[IBIS Ver]   4.2
[File Name]  stm32f2_lqfp176.ibs
[File Rev]   1.0
[Date]   31-Aug-2011
[Source]   STMicroelectronics NV
[Notes]   The I/O models have been made by simulation and qualified
   with recomandation of QualityIBIS flow.
   Some Models, library and pin names may be modified.
   Details of modified names can be found below.
ORIGINAL NAME   ::  MODIFIED NAME   :: COMMENTS(if any)
IO8USB_LSFS_OTG_FT  ::  IO8USB_LSFS_OTG_FT_USB   :: Model in USB mode.
IO8USB_LSFS_OTG_FT  ::  IO8USB_LSFS_OTG_FT_NON_USB_DNV33  :: Model in other than USB mode & pad pin = DNV33
IO8USB_LSFS_OTG_FT  ::  IO8USB_LSFS_OTG_FT_NON_USB_DPV33  :: Model in other than USB mode & pad pin = DPV33
[Disclaimer] These IBIS models are the proprietary information of
   STMicroelectronics and are disclosed to users solely for
   modeling and simulation purposes. No further license is
   implied. All warranties express, implied, or statutory,
   including any implied warranty of fitness for a particular
   purpose or implied warranty against infringement, are
   hereby disclaimed. STMicroelectronics reserves the right
   to change the IBIS models at any time and without notice.
[Copyright]  (c) STMicroelectronics
   All rights reserved. Reproduction in whole or part is prohibited
   without the written consent of the copyright holder.
[Component]  STM32F2_LQFP176
[Manufacturer] STMicroelectronics NV
[Package]
| variable   typ   min   max
R_pkg   0.000mOhm   0.000mOhm   0.000mOhm
L_pkg   0.000nH   0.000nH   0.000nH
C_pkg   0.000pF   0.000pF   0.000pF
[Pin]   signal_name   model_name
1 PE2 IO8PROG2M25M50M100M_ARSUDQ_FT
2 PE3 IO8PROG2M25M50M100M_ARSUDQ_FT
3 PE4 IO8PROG2M25M50M100M_ARSUDQ_FT
4 PE5 IO8PROG2M25M50M100M_ARSUDQ_FT
5 PE6 IO8PROG2M25M50M100M_ARSUDQ_FT
|6 VBAT VDD33IOSWCO_MOSSWI_FT
7 PI8 IO8PROG2M25M50M100M_ARSUDQ_FT_V33
8 PC13 IO8PROG2M25M50M100M_ARWSUDQ_FT_V33
9 PC14 IO8PROG2M25M50M100M_ARWSUDQ_FT
10 PC15 IO8PROG2M25M50M100M_ARSUDQ_FT
11 PI9  IO8PROG2M25M50M100M_ARSUDQ_FT
12 PI10 IO8PROG2M25M50M100M_ARSUDQ_FT
13 PI11 IO8PROG2M25M50M100M_ARSUDQ_FT
|14 VSS_13 VSSIOCO
|15 VDD_13 VDD33IOCO
16 PF0 IO8PROG2M25M50M100M_ARSUDQ_FT
17 PF1 IO8PROG2M25M50M100M_ARSUDQ_FT
18 PF2 IO8PROG2M25M50M100M_ARSUDQ_FT
19 PF3 IO8PROG2M25M50M100M_ARSUDQ_FT
20 PF4 IO8PROG2M25M50M100M_ARSUDQ_FT
21 PF5 IO8PROG2M25M50M100M_ARSUDQ_FT
|22 VSS_5 VSSIOCO
|23 VDD_5 VDD33IOCO
24 PF6 IO8PROG2M25M50M100M_ARSUDQ_FT
25 PF7 IO8PROG2M25M50M100M_ARSUDQ_FT
26 PF8 IO8PROG2M25M50M100M_ARSUDQ_FT
27 PF9  IO8PROG2M25M50M100M_AR3WSUDQ_FT
28 PF10 IO8PROG2M25M50M100M_ARSUDQ_FT
29 PH0 IO8PROG2M25M50M100M_ARSUDQ_FT
30 PH1 IO8PROG2M25M50M100M_ARSUDQ_FT
|31 NRST RESET
32 PC0 IO8PROG2M25M50M100M_AR3WSUDQ_FT
33 PC1 IO8PROG2M25M50M100M_AR3WSUDQ_FT
34 PC2 IO8PROG2M25M50M100M_AR3WSUDQ_FT
35 PC3 IO8PROG2M25M50M100M_AR3WSUDQ_FT
|36 VDD_12 VDD33IOCO_VSSIOCO_MOSSWI_FT
|37 VSSA VSSCO
|38 VREF+ VDD33CO
|39 VDDA VDD33CO
40 PA0 IO8PROG2M25M50M100M_AR3WSUDQ_FT_V33
41 PA1 IO8PROG2M25M50M100M_AR3WSUDQ_FT
42 PA2 IO8PROG2M25M50M100M_AR3WSUDQ_FT
43 PH2 IO8PROG2M25M50M100M_AR3WSUDQ_FT
44 PH3 IO8PROG2M25M50M100M_AR3WSUDQ_FT
45 PH4 IO8PROG2M25M50M100M_AR3WSUDQ_FT
46 PH5 IO8PROG2M25M50M100M_AR3WSUDQ_FT
47 PA3 IO8PROG2M25M50M100M_AR3WSUDQ_FT
|48 VSS_4 VSSIOCO
|49 VDD_4 VDD33IOCO
50 PA4 IO8PROG2M25M50M100M_AR3WSUDQ_FT
51 PA5 IO8PROG2M25M50M100M_AR3WSUDQ_FT
52 PA6 IO8PROG2M25M50M100M_AR3WSUDQ_FT
53 PA7 IO8PROG2M25M50M100M_AR3WSUDQ_FT
54 PC4 IO8PROG2M25M50M100M_AR3WSUDQ_FT
55 PC5 IO8PROG2M25M50M100M_AR3WSUDQ_FT
56 PB0 IO8PROG2M25M50M100M_AR3WSUDQ_FT
57 PB1 IO8PROG2M25M50M100M_AR3WSUDQ_FT
58 PB2 IO8PROG2M25M50M100M_AR3WSUDQ_FT
59 PF11 IO8PROG2M25M50M100M_ARSUDQ_FT
60 PF12 IO8PROG2M25M50M100M_ARSUDQ_FT
|61 VSS_6 VSSIOCO
|62 VDD_6 VDD33IOCO
63 PF13 IO8PROG2M25M50M100M_ARSUDQ_FT
64 PF14 IO8PROG2M25M50M100M_ARSUDQ_FT
65 PF15 IO8PROG2M25M50M100M_ARSUDQ_FT
66 PG0 IO8PROG2M25M50M100M_ARSUDQ_FT
67 PG1 IO8PROG2M25M50M100M_ARSUDQ_FT
68 PE7 IO8PROG2M25M50M100M_ARSUDQ_FT
69 PE8 IO8PROG2M25M50M100M_ARSUDQ_FT
70 PE9 IO8PROG2M25M50M100M_ARSUDQ_FT
|71 VSS_7 VSSIOCO
|72 VDD_7 VDD33IOCO
73 PE10 IO8PROG2M25M50M100M_ARSUDQ_FT
74 PE11 IO8PROG2M25M50M100M_ARSUDQ_FT
75 PE12 IO8PROG2M25M50M100M_ARSUDQ_FT
76 PE13 IO8PROG2M25M50M100M_ARSUDQ_FT
77 PE14 IO8PROG2M25M50M100M_ARSUDQ_FT
78 PE15 IO8PROG2M25M50M100M_ARSUDQ_FT
79 PB10 IO8PROG2M25M50M100M_ARSUDQ_I2CIN_FT
80 PB11 IO8PROG2M25M50M100M_ARSUDQ_I2CIN_FT
|81 VCAP_1
|82 VDD_1 VDD33IOCO
83 PH6 IO8PROG2M25M50M100M_ARSUDQ_FT
84 PH7 IO8PROG2M25M50M100M_ARSUDQ_FT
85 PH8 IO8PROG2M25M50M100M_ARSUDQ_FT
86 PH9 IO8PROG2M25M50M100M_ARSUDQ_FT
87 PH10 IO8PROG2M25M50M100M_ARSUDQ_FT
88 PH11 IO8PROG2M25M50M100M_ARSUDQ_FT
89 PH12 IO8PROG2M25M50M100M_ARSUDQ_FT
|90 VSS_14 VSSIOCO
|91 VDD_14 VDD33IOCO
92 PB12 IO8USB_ID_OTG_FT
93 PB13 IO8USB_VBUS_OTG_FT
94 PB14 IO8USB_LSFS_OTG_FT_USB
|94 PB14 IO8USB_LSFS_OTG_FT_NON_USB_DNV33
95 PB15 IO8USB_LSFS_OTG_FT_USB
|95 PB15 IO8USB_LSFS_OTG_FT_NON_USB_DPV3394
96 PD8 IO8PROG2M25M50M100M_ARSUDQ_FT
97 PD9 IO8PROG2M25M50M100M_ARSUDQ_FT
98 PD10 IO8PROG2M25M50M100M_ARSUDQ_FT
99 PD11 IO8PROG2M25M50M100M_ARSUDQ_FT
100 PD12 IO8PROG2M25M50M100M_ARSUDQ_FT
101 PD13 IO8PROG2M25M50M100M_ARSUDQ_FT
|102 VSS_8 VSSIOCO
|103 VDD_8 VDD33IOCO
104 PD14 IO8PROG2M25M50M100M_ARSUDQ_FT
105 PD15 IO8PROG2M25M50M100M_ARSUDQ_FT
106 PG2 IO8PROG2M25M50M100M_ARSUDQ_FT
107 PG3 IO8PROG2M25M50M100M_ARSUDQ_FT
108 PG4 IO8PROG2M25M50M100M_ARSUDQ_FT
109 PG5 IO8PROG2M25M50M100M_ARSUDQ_FT
110 PG6 IO8PROG2M25M50M100M_ARSUDQ_FT
111 PG7 IO8PROG2M25M50M100M_ARSUDQ_FT
112 PG8 IO8PROG2M25M50M100M_ARSUDQ_FT
|113 VSS_9 VSSIOCO
|114 VDD_9 VDD33IOCO
115 PC6 IO8PROG2M25M50M100M_ARSUDQ_FT
116 PC7 IO8PROG2M25M50M100M_ARSUDQ_FT
117 PC8 IO8PROG2M25M50M100M_ARSUDQ_FT
118 PC9 IO8PROG2M25M50M100M_ARSUDQ_I2CIN_FT
119 PA8 IO8PROG2M25M50M100M_ARSUDQ_I2CIN_FT
120 PA9 IO8USB_VBUS_OTG_FT
121 PA10 IO8USB_ID_OTG_FT
|122 PA11 IO8USB_LSFS_OTG_FT_USB
122 PA11 IO8USB_LSFS_OTG_FT_NON_USB_DNV33
|123 PA12 IO8USB_LSFS_OTG_FT_USB
123 PA12 IO8USB_LSFS_OTG_FT_NON_USB_DPV33
124 PA13 IO8PROG2M25M50M100M_ARSUDQ_FT
|125 VCAP_2
|126 VSS_2 VSSIOCO
|127 VDD_2 VDD33IOCO
128 PH13 IO8PROG2M25M50M100M_ARSUDQ_FT
129 PH14 IO8PROG2M25M50M100M_ARSUDQ_FT
130 PH15 IO8PROG2M25M50M100M_ARSUDQ_FT
131 PI0 IO8PROG2M25M50M100M_ARSUDQ_FT
132 PI1 IO8PROG2M25M50M100M_ARSUDQ_FT
133 PI2 IO8PROG2M25M50M100M_ARSUDQ_FT
134 PI3 IO8PROG2M25M50M100M_ARSUDQ_FT
|135 VSS_15 VSSIOCO
|136 VDD_15 VDD33IOCO
137 PA14 IO8PROG2M25M50M100M_ARSUDQ_FT
138 PA15 IO8PROG2M25M50M100M_AR3WSUDQ_FT
139 PC10 IO8PROG2M25M50M100M_ARSUDQ_FT
140 PC11 IO8PROG2M25M50M100M_ARSUDQ_FT
141 PC12 IO8PROG2M25M50M100M_ARSUDQ_FT
142 PD0 IO8PROG2M25M50M100M_ARSUDQ_FT
143 PD1 IO8PROG2M25M50M100M_ARSUDQ_FT
144 PD2 IO8PROG2M25M50M100M_ARSUDQ_FT
145 PD3 IO8PROG2M25M50M100M_ARSUDQ_FT
146 PD4 IO8PROG2M25M50M100M_ARSUDQ_FT
147 PD5 IO8PROG2M25M50M100M_ARSUDQ_FT
|148 VSS_10 VSSIOCO
|149 VDD_10 VDD33IOCO
150 PD6 IO8PROG2M25M50M100M_ARSUDQ_FT
151 PD7 IO8PROG2M25M50M100M_ARSUDQ_FT
152 PG9 IO8PROG2M25M50M100M_ARSUDQ_FT
153 PG10 IO8PROG2M25M50M100M_ARSUDQ_FT
154 PG11 IO8PROG2M25M50M100M_ARSUDQ_FT
155 PG12 IO8PROG2M25M50M100M_ARSUDQ_FT
156 PG13 IO8PROG2M25M50M100M_ARSUDQ_FT
157 PG14 IO8PROG2M25M50M100M_ARSUDQ_FT
|158 VSS_11 VSSIOCO
|159 VDD_11 VDD33IOCO
160 PG15 IO8PROG2M25M50M100M_ARSUDQ_FT
161 PB3 IO8PROG2M25M50M100M_ARSUDQ_FT
162 PB4 IO8PROG2M25M50M100M_ARSUDQ_FT
163 PB5 IO8PROG2M25M50M100M_AR3WSUDQ_FT
164 PB6 IO8PROG2M25M50M100M_ARSUDQ_I2CIN_FT
165 PB7 IO8PROG2M25M50M100M_ARSUDQ_I2CIN_FT
166 BOOT0 VPP_TEST_HV
167 PB8 IO8PROG2M25M50M100M_ARSUDQ_I2CIN_FT
168 PB9 IO8PROG2M25M50M100M_ARSUDQ_I2CIN_FT
169 PE0 IO8PROG2M25M50M100M_ARSUDQ_FT
170 PE1 IO8PROG2M25M50M100M_ARSUDQ_FT
|171 VSS VSSIOCO
|172 VDD_3 VDD33IOCO
173 PI4 IO8PROG2M25M50M100M_ARSUDQ_FT
174 PI5 IO8PROG2M25M50M100M_ARSUDQ_FT
175 PI6 IO8PROG2M25M50M100M_ARSUDQ_FT
176 PI7 IO8PROG2M25M50M100M_ARSUDQ_FT
[Diff Pin]  inv_pin   vdiff tdelay_typ tdelay_min tdelay_max
94 95 200mV 0  0 0
122 123 200mV 0  0 0
[Model Selector] IO8PROG2M25M50M100M_ARSUDQ_FT_V33
IO8PROG2M25M50M100M_ARSUDQ_DRV_V33_00   DRIVER MODEL  : SPEEDAV33=0 SPEEDBV33=0
IO8PROG2M25M50M100M_ARSUDQ_DRV_V33_01   DRIVER MODEL  : SPEEDAV33=0 SPEEDBV33=1
IO8PROG2M25M50M100M_ARSUDQ_DRV_V33_10   DRIVER MODEL  : SPEEDAV33=1 SPEEDBV33=0
IO8PROG2M25M50M100M_ARSUDQ_DRV_V33_11   DRIVER MODEL  : SPEEDAV33=1 SPEEDBV33=1
IO8PROG2M25M50M100M_ARSUDQ_RCV_V33_0   CMOS RECIEVER : ENHYSV33=0  OUTPUT=ZIV33
IO8PROG2M25M50M100M_ARSUDQ_RCV_V33_0_T   TTL  RECIEVER : ENHYSV33=0  OUTPUT=ZIV33
IO8PROG2M25M50M100M_ARSUDQ_RCV_V33_1   CMOS RECIEVER : ENHYSV33=1  OUTPUT=ZIV33
IO8PROG2M25M50M100M_ARSUDQ_RCV_V33_1_T   TTL  RECIEVER : ENHYSV33=1  OUTPUT=ZIV33
[Model Selector] IO8PROG2M25M50M100M_AR3WSUDQ_FT_V33
IO8PROG2M25M50M100M_AR3WSUDQ_DRV_V33_00   DRIVER MODEL  : SPEEDAV33=0 SPEEDBV33=0
IO8PROG2M25M50M100M_AR3WSUDQ_DRV_V33_01   DRIVER MODEL  : SPEEDAV33=0 SPEEDBV33=1
IO8PROG2M25M50M100M_AR3WSUDQ_DRV_V33_10   DRIVER MODEL  : SPEEDAV33=1 SPEEDBV33=0
IO8PROG2M25M50M100M_AR3WSUDQ_DRV_V33_11   DRIVER MODEL  : SPEEDAV33=1 SPEEDBV33=1
IO8PROG2M25M50M100M_AR3WSUDQ_RCV_V33_0   CMOS RECIEVER : ENHYSV33=0  OUTPUT=ZIV33
IO8PROG2M25M50M100M_AR3WSUDQ_RCV_V33_0_T  TTL  RECIEVER : ENHYSV33=0  OUTPUT=ZIV33
IO8PROG2M25M50M100M_AR3WSUDQ_RCV_V33_1   CMOS RECIEVER : ENHYSV33=1  OUTPUT=ZIV33
IO8PROG2M25M50M100M_AR3WSUDQ_RCV_V33_1_T  TTL  RECIEVER : ENHYSV33=1  OUTPUT=ZIV33
[Model Selector] IO8PROG2M25M50M100M_AR3WSUDQ_FT
IO8PROG2M25M50M100M_AR3WSUDQ_FT_DRV_00   DRIVER MODEL  : SPEEDAV12=0 SPEEDBV12=0
IO8PROG2M25M50M100M_AR3WSUDQ_FT_DRV_01   DRIVER MODEL  : SPEEDAV12=0 SPEEDBV12=1
IO8PROG2M25M50M100M_AR3WSUDQ_FT_DRV_10   DRIVER MODEL  : SPEEDAV12=1 SPEEDBV12=0
IO8PROG2M25M50M100M_AR3WSUDQ_FT_DRV_11   DRIVER MODEL  : SPEEDAV12=1 SPEEDBV12=1
IO8PROG2M25M50M100M_AR3WSUDQ_FT_RCV_00   CMOS RECIEVER : ENHYSV12=0  OUTPUT=ZIV12
IO8PROG2M25M50M100M_AR3WSUDQ_FT_RCV_00_T  TTL  RECIEVER : ENHYSV12=0  OUTPUT=ZIV12
IO8PROG2M25M50M100M_AR3WSUDQ_FT_RCV_01   CMOS RECIEVER : ENHYSV12=0  OUTPUT=ZIV33
IO8PROG2M25M50M100M_AR3WSUDQ_FT_RCV_01_T  TTL  RECIEVER : ENHYSV12=0  OUTPUT=ZIV33
IO8PROG2M25M50M100M_AR3WSUDQ_FT_RCV_10   CMOS RECIEVER : ENHYSV12=1  OUTPUT=ZIV12
IO8PROG2M25M50M100M_AR3WSUDQ_FT_RCV_10_T  TTL  RECIEVER : ENHYSV12=1  OUTPUT=ZIV12
IO8PROG2M25M50M100M_AR3WSUDQ_FT_RCV_11   CMOS RECIEVER : ENHYSV12=1  OUTPUT=ZIV33
IO8PROG2M25M50M100M_AR3WSUDQ_FT_RCV_11_T  TTL  RECIEVER : ENHYSV12=1  OUTPUT=ZIV33
[Model Selector] IO8PROG2M25M50M100M_ARSUDQ_FT
IO8PROG2M25M50M100M_ARSUDQ_FT_DRV_00   DRIVER MODEL  : SPEEDAV12=0 SPEEDBV12=0
IO8PROG2M25M50M100M_ARSUDQ_FT_DRV_01   DRIVER MODEL  : SPEEDAV12=0 SPEEDBV12=1
IO8PROG2M25M50M100M_ARSUDQ_FT_DRV_10   DRIVER MODEL  : SPEEDAV12=1 SPEEDBV12=0
IO8PROG2M25M50M100M_ARSUDQ_FT_DRV_11   DRIVER MODEL  : SPEEDAV12=1 SPEEDBV12=1
IO8PROG2M25M50M100M_ARSUDQ_FT_RCV_00   CMOS RECIEVER : ENHYSV12=0  OUTPUT=ZIV12
IO8PROG2M25M50M100M_ARSUDQ_FT_RCV_00_T   TTL  RECIEVER : ENHYSV12=0  OUTPUT=ZIV12
IO8PROG2M25M50M100M_ARSUDQ_FT_RCV_01   CMOS RECIEVER : ENHYSV12=0  OUTPUT=ZIV33
IO8PROG2M25M50M100M_ARSUDQ_FT_RCV_01_T   TTL  RECIEVER : ENHYSV12=0  OUTPUT=ZIV33
IO8PROG2M25M50M100M_ARSUDQ_FT_RCV_10   CMOS RECIEVER : ENHYSV12=1  OUTPUT=ZIV12
IO8PROG2M25M50M100M_ARSUDQ_FT_RCV_10_T   TTL  RECIEVER : ENHYSV12=1  OUTPUT=ZIV12
IO8PROG2M25M50M100M_ARSUDQ_FT_RCV_11   CMOS RECIEVER : ENHYSV12=1  OUTPUT=ZIV33
IO8PROG2M25M50M100M_ARSUDQ_FT_RCV_11_T   TTL  RECIEVER : ENHYSV12=1  OUTPUT=ZIV33
[Model Selector] IO8PROG2M25M50M100M_ARSUDQ_I2CIN_FT
IO8PROG2M25M50M100M_ARSUDQ_I2CIN_DRV_00   DRIVER MODEL  : SPEEDAV12=0 SPEEDBV12=0
IO8PROG2M25M50M100M_ARSUDQ_I2CIN_DRV_01   DRIVER MODEL  : SPEEDAV12=0 SPEEDBV12=1
IO8PROG2M25M50M100M_ARSUDQ_I2CIN_DRV_10   DRIVER MODEL  : SPEEDAV12=1 SPEEDBV12=0
IO8PROG2M25M50M100M_ARSUDQ_I2CIN_DRV_11   DRIVER MODEL  : SPEEDAV12=1 SPEEDBV12=1
IO8PROG2M25M50M100M_I2CIN_RCV_ZII2C_00   CMOS RECIEVER : TESTI2CV12=0  HSFSV12=0
IO8PROG2M25M50M100M_I2CIN_RCV_ZII2C_00_T   TTL  RECIEVER : TESTI2CV12=0  HSFSV12=0
IO8PROG2M25M50M100M_I2CIN_RCV_ZII2C_01   CMOS RECIEVER : TESTI2CV12=0  HSFSV12=1
IO8PROG2M25M50M100M_I2CIN_RCV_ZII2C_01_T   TTL  RECIEVER : TESTI2CV12=0  HSFSV12=1
IO8PROG2M25M50M100M_I2CIN_RCV_ZII2C_10   CMOS RECIEVER : TESTI2CV12=1  HSFSV12=0
IO8PROG2M25M50M100M_I2CIN_RCV_ZII2C_10_T   TTL  RECIEVER : TESTI2CV12=1  HSFSV12=0
IO8PROG2M25M50M100M_I2CIN_RCV_ZII2C_11   CMOS RECIEVER : TESTI2CV12=1  HSFSV12=1
IO8PROG2M25M50M100M_I2CIN_RCV_ZII2C_11_T   TTL  RECIEVER : TESTI2CV12=1  HSFSV12=1
IO8PROG2M25M50M100M_I2CIN_RCV_ZIV12_0   CMOS RECIEVER : ENHYSV12=0  OUTPUT=ZIV12
IO8PROG2M25M50M100M_I2CIN_RCV_ZIV12_0_T   TTL  RECIEVER : ENHYSV12=0  OUTPUT=ZIV12
IO8PROG2M25M50M100M_I2CIN_RCV_ZIV12_1   CMOS RECIEVER : ENHYSV12=1  OUTPUT=ZIV12
IO8PROG2M25M50M100M_I2CIN_RCV_ZIV12_1_T   TTL  RECIEVER : ENHYSV12=1  OUTPUT=ZIV12
IO8PROG2M25M50M100M_I2CIN_RCV_ZIV33_0   CMOS RECIEVER : ENHYSV12=0  OUTPUT=ZIV33
IO8PROG2M25M50M100M_I2CIN_RCV_ZIV33_0_T   TTL  RECIEVER : ENHYSV12=0  OUTPUT=ZIV33
IO8PROG2M25M50M100M_I2CIN_RCV_ZIV33_1   CMOS RECIEVER : ENHYSV12=1  OUTPUT=ZIV33
IO8PROG2M25M50M100M_I2CIN_RCV_ZIV33_1_T   TTL  RECIEVER : ENHYSV12=1  OUTPUT=ZIV33
[Model Selector] IO8PROG2M25M50M100M_ARWSUDQ_FT_V33
IO8PROG2M25M50M100M_ARWSUDQ_DRV_V33_00   DRIVER MODEL  : SPEEDAV33=0 SPEEDBV33=0
IO8PROG2M25M50M100M_ARWSUDQ_DRV_V33_01   DRIVER MODEL  : SPEEDAV33=0 SPEEDBV33=1
IO8PROG2M25M50M100M_ARWSUDQ_DRV_V33_10   DRIVER MODEL  : SPEEDAV33=1 SPEEDBV33=0
IO8PROG2M25M50M100M_ARWSUDQ_DRV_V33_11   DRIVER MODEL  : SPEEDAV33=1 SPEEDBV33=1
IO8PROG2M25M50M100M_ARWSUDQ_RCV_V33_0   CMOS RECIEVER : ENHYSV33=0  OUTPUT=ZIV33
IO8PROG2M25M50M100M_ARWSUDQ_RCV_V33_0_T   TTL  RECIEVER : ENHYSV33=0  OUTPUT=ZIV33
IO8PROG2M25M50M100M_ARWSUDQ_RCV_V33_1   CMOS RECIEVER : ENHYSV33=1  OUTPUT=ZIV33
IO8PROG2M25M50M100M_ARWSUDQ_RCV_V33_1_T   TTL  RECIEVER : ENHYSV33=1  OUTPUT=ZIV33
[Model Selector] IO8PROG2M25M50M100M_ARWSUDQ_FT
IO8PROG2M25M50M100M_ARWSUDQ_FT_DRV_00   DRIVER MODEL  : SPEEDAV12=0 SPEEDBV12=0
IO8PROG2M25M50M100M_ARWSUDQ_FT_DRV_01   DRIVER MODEL  : SPEEDAV12=0 SPEEDBV12=1
IO8PROG2M25M50M100M_ARWSUDQ_FT_DRV_10   DRIVER MODEL  : SPEEDAV12=1 SPEEDBV12=0
IO8PROG2M25M50M100M_ARWSUDQ_FT_DRV_11   DRIVER MODEL  : SPEEDAV12=1 SPEEDBV12=1
IO8PROG2M25M50M100M_ARWSUDQ_FT_RCV_00   CMOS RECIEVER : ENHYSV12=0  OUTPUT=ZIV12
IO8PROG2M25M50M100M_ARWSUDQ_FT_RCV_00_T   TTL  RECIEVER : ENHYSV12=0  OUTPUT=ZIV12
IO8PROG2M25M50M100M_ARWSUDQ_FT_RCV_01   CMOS RECIEVER : ENHYSV12=0  OUTPUT=ZIV33
IO8PROG2M25M50M100M_ARWSUDQ_FT_RCV_01_T   TTL  RECIEVER : ENHYSV12=0  OUTPUT=ZIV33
IO8PROG2M25M50M100M_ARWSUDQ_FT_RCV_10   CMOS RECIEVER : ENHYSV12=1  OUTPUT=ZIV12
IO8PROG2M25M50M100M_ARWSUDQ_FT_RCV_10_T   TTL  RECIEVER : ENHYSV12=1  OUTPUT=ZIV12
IO8PROG2M25M50M100M_ARWSUDQ_FT_RCV_11   CMOS RECIEVER : ENHYSV12=1  OUTPUT=ZIV33
IO8PROG2M25M50M100M_ARWSUDQ_FT_RCV_11_T   TTL  RECIEVER : ENHYSV12=1  OUTPUT=ZIV33
[Model Selector] IO8USB_ID_OTG_FT
IO8USB_ID_OTG_FT_DRV_00   DRIVER MODEL  : SPEEDAV12=0 SPEEDBV12=0
IO8USB_ID_OTG_FT_DRV_01   DRIVER MODEL  : SPEEDAV12=0 SPEEDBV12=1
IO8USB_ID_OTG_FT_DRV_10   DRIVER MODEL  : SPEEDAV12=1 SPEEDBV12=0
IO8USB_ID_OTG_FT_DRV_11   DRIVER MODEL  : SPEEDAV12=1 SPEEDBV12=1
IO8USB_ID_OTG_FT_RCV_00   CMOS RECIEVER : ENHYSV12=0  OUTPUT=ZIV12
IO8USB_ID_OTG_FT_RCV_00_T   TTL  RECIEVER : ENHYSV12=0  OUTPUT=ZIV12
IO8USB_ID_OTG_FT_RCV_01   CMOS RECIEVER : ENHYSV12=0  OUTPUT=ZIV33
IO8USB_ID_OTG_FT_RCV_01_T   TTL  RECIEVER : ENHYSV12=0  OUTPUT=ZIV33
IO8USB_ID_OTG_FT_RCV_10   CMOS RECIEVER : ENHYSV12=1  OUTPUT=ZIV12
IO8USB_ID_OTG_FT_RCV_10_T   TTL  RECIEVER : ENHYSV12=1  OUTPUT=ZIV12
IO8USB_ID_OTG_FT_RCV_11   CMOS RECIEVER : ENHYSV12=1  OUTPUT=ZIV33
IO8USB_ID_OTG_FT_RCV_11_T   TTL  RECIEVER : ENHYSV12=1  OUTPUT=ZIV33
[Model Selector] IO8USB_LSFS_OTG_FT_USB
IO8USB_LSFS_OTG_FT_DRV_USB_0   DRIVER : USBLSFSV12=0 ENUSBV12=0
IO8USB_LSFS_OTG_FT_DRV_USB_1   DRIVER : USBLSFSV12=1 ENUSBV12=0
IO8USB_LSFS_OTG_FT_RCV_USB   USB  RECIEVER : ENHYSV12=1  OUTPUT=USBZIV12
[Model Selector] IO8USB_LSFS_OTG_FT_NON_USB_DNV33
IO8USB_LSFS_OTG_FT_DRV_IO8_DNV33_00   DRIVER : SPEEDAV12=0 SPEEDBV12=0 ENUSBV12=1
IO8USB_LSFS_OTG_FT_DRV_IO8_DNV33_01   DRIVER : SPEEDAV12=0 SPEEDBV12=1 ENUSBV12=1
IO8USB_LSFS_OTG_FT_DRV_IO8_DNV33_10   DRIVER : SPEEDAV12=1 SPEEDBV12=0 ENUSBV12=1
IO8USB_LSFS_OTG_FT_DRV_IO8_DNV33_11   DRIVER : SPEEDAV12=1 SPEEDBV12=1 ENUSBV12=1
IO8USB_LSFS_OTG_FT_RCV_IO8_ZINV12_0   CMOS RECIEVER : ENHYSV12=0  OUTPUT=ZIV12
IO8USB_LSFS_OTG_FT_RCV_IO8_ZINV12_0_T  TTL  RECIEVER : ENHYSV12=0  OUTPUT=ZIV12
IO8USB_LSFS_OTG_FT_RCV_IO8_ZINV12_1   CMOS RECIEVER : ENHYSV12=1  OUTPUT=ZIV12
IO8USB_LSFS_OTG_FT_RCV_IO8_ZINV12_1_T  TTL  RECIEVER : ENHYSV12=1  OUTPUT=ZIV12
IO8USB_LSFS_OTG_FT_RCV_IO8_ZINV33_0   CMOS RECIEVER : ENHYSV12=0  OUTPUT=ZIV33
IO8USB_LSFS_OTG_FT_RCV_IO8_ZINV33_0_T  TTL  RECIEVER : ENHYSV12=0  OUTPUT=ZIV33
IO8USB_LSFS_OTG_FT_RCV_IO8_ZINV33_1   CMOS RECIEVER : ENHYSV12=1  OUTPUT=ZIV33
IO8USB_LSFS_OTG_FT_RCV_IO8_ZINV33_1_T  TTL  RECIEVER : ENHYSV12=1  OUTPUT=ZIV33
[Model Selector] IO8USB_LSFS_OTG_FT_NON_USB_DPV33
IO8USB_LSFS_OTG_FT_DRV_IO8_DPV33_00   DRIVER : SPEEDAV12=0 SPEEDBV12=0 ENUSBV12=1
IO8USB_LSFS_OTG_FT_DRV_IO8_DPV33_01   DRIVER : SPEEDAV12=0 SPEEDBV12=1 ENUSBV12=1
IO8USB_LSFS_OTG_FT_DRV_IO8_DPV33_10   DRIVER : SPEEDAV12=1 SPEEDBV12=0 ENUSBV12=1
IO8USB_LSFS_OTG_FT_DRV_IO8_DPV33_11   DRIVER : SPEEDAV12=1 SPEEDBV12=1 ENUSBV12=1
IO8USB_LSFS_OTG_FT_RCV_IO8_ZIPV12_0   CMOS RECIEVER : ENHYSV12=0  OUTPUT=ZIV12
IO8USB_LSFS_OTG_FT_RCV_IO8_ZIPV12_0_T  TTL  RECIEVER : ENHYSV12=0  OUTPUT=ZIV12
IO8USB_LSFS_OTG_FT_RCV_IO8_ZIPV12_1   CMOS RECIEVER : ENHYSV12=1  OUTPUT=ZIV12
IO8USB_LSFS_OTG_FT_RCV_IO8_ZIPV12_1_T  TTL  RECIEVER : ENHYSV12=1  OUTPUT=ZIV12
IO8USB_LSFS_OTG_FT_RCV_IO8_ZIPV33_0   CMOS RECIEVER : ENHYSV12=0  OUTPUT=ZIV33
IO8USB_LSFS_OTG_FT_RCV_IO8_ZIPV33_0_T  TTL  RECIEVER : ENHYSV12=0  OUTPUT=ZIV33
IO8USB_LSFS_OTG_FT_RCV_IO8_ZIPV33_1   CMOS RECIEVER : ENHYSV12=1  OUTPUT=ZIV33
IO8USB_LSFS_OTG_FT_RCV_IO8_ZIPV33_1_T  TTL  RECIEVER : ENHYSV12=1  OUTPUT=ZIV33
[Model Selector] IO8USB_VBUS_OTG_FT
IO8USB_VBUS_OTG_FT_DRV_00   DRIVER MODEL  : SPEEDAV12=0 SPEEDBV12=0
IO8USB_VBUS_OTG_FT_DRV_01   DRIVER MODEL  : SPEEDAV12=0 SPEEDBV12=1
IO8USB_VBUS_OTG_FT_DRV_10   DRIVER MODEL  : SPEEDAV12=1 SPEEDBV12=0
IO8USB_VBUS_OTG_FT_DRV_11   DRIVER MODEL  : SPEEDAV12=1 SPEEDBV12=1
IO8USB_VBUS_OTG_FT_RCV_00   CMOS RECIEVER : ENHYSV12=0  OUTPUT=ZIV12
IO8USB_VBUS_OTG_FT_RCV_00_T   TTL  RECIEVER : ENHYSV12=0  OUTPUT=ZIV12
IO8USB_VBUS_OTG_FT_RCV_01   CMOS RECIEVER : ENHYSV12=0  OUTPUT=ZIV33
IO8USB_VBUS_OTG_FT_RCV_01_T   TTL  RECIEVER : ENHYSV12=0  OUTPUT=ZIV33
IO8USB_VBUS_OTG_FT_RCV_10   CMOS RECIEVER : ENHYSV12=1  OUTPUT=ZIV12
IO8USB_VBUS_OTG_FT_RCV_10_T   TTL  RECIEVER : ENHYSV12=1  OUTPUT=ZIV12
IO8USB_VBUS_OTG_FT_RCV_11   CMOS RECIEVER : ENHYSV12=1  OUTPUT=ZIV33
IO8USB_VBUS_OTG_FT_RCV_11_T   TTL  RECIEVER : ENHYSV12=1  OUTPUT=ZIV33
[Model Selector] VPP_TEST_HV
VPP_TEST_HV_00   CMOS RECIEVER : ENHYSV12=0  OUTPUT=ZIV12
VPP_TEST_HV_00_T   TTL  RECIEVER : ENHYSV12=0  OUTPUT=ZIV12
VPP_TEST_HV_01   CMOS RECIEVER : ENHYSV12=0  OUTPUT=ZIV33
VPP_TEST_HV_01_T   TTL  RECIEVER : ENHYSV12=0  OUTPUT=ZIV33
VPP_TEST_HV_10   CMOS RECIEVER : ENHYSV12=1  OUTPUT=ZIV12
VPP_TEST_HV_10_T   TTL  RECIEVER : ENHYSV12=1  OUTPUT=ZIV12
VPP_TEST_HV_11   CMOS RECIEVER : ENHYSV12=1  OUTPUT=ZIV33
VPP_TEST_HV_11_T   TTL  RECIEVER : ENHYSV12=1  OUTPUT=ZIV33
| Models and submodels in the file (139): IO8PROG2M25M50M100M_AR3WSUDQ_DRV_V33_00 (3-state), IO8PROG2M25M50M100M_AR3WSUDQ_DRV_V33_01 (3-state), IO8PROG2M25M50M100M_AR3WSUDQ_DRV_V33_10 (3-state), IO8PROG2M25M50M100M_AR3WSUDQ_DRV_V33_11 (3-state), IO8PROG2M25M50M100M_AR3WSUDQ_FT_DRV_00 (3-state), IO8PROG2M25M50M100M_AR3WSUDQ_FT_DRV_01 (3-state), IO8PROG2M25M50M100M_AR3WSUDQ_FT_DRV_10 (3-state), IO8PROG2M25M50M100M_AR3WSUDQ_FT_DRV_11 (3-state), IO8PROG2M25M50M100M_AR3WSUDQ_FT_RCV_00 (Input), IO8PROG2M25M50M100M_AR3WSUDQ_FT_RCV_00_T (Input), IO8PROG2M25M50M100M_AR3WSUDQ_FT_RCV_01 (Input), IO8PROG2M25M50M100M_AR3WSUDQ_FT_RCV_01_T (Input), IO8PROG2M25M50M100M_AR3WSUDQ_FT_RCV_10 (Input), IO8PROG2M25M50M100M_AR3WSUDQ_FT_RCV_10_T (Input), IO8PROG2M25M50M100M_AR3WSUDQ_FT_RCV_11 (Input), IO8PROG2M25M50M100M_AR3WSUDQ_FT_RCV_11_T (Input), IO8PROG2M25M50M100M_AR3WSUDQ_RCV_V33_0 (Input), IO8PROG2M25M50M100M_AR3WSUDQ_RCV_V33_0_T (Input), IO8PROG2M25M50M100M_AR3WSUDQ_RCV_V33_1 (Input), IO8PROG2M25M50M100M_AR3WSUDQ_RCV_V33_1_T (Input), IO8PROG2M25M50M100M_ARSUDQ_FT_DRV_00 (3-state), IO8PROG2M25M50M100M_ARSUDQ_FT_DRV_01 (3-state), IO8PROG2M25M50M100M_ARSUDQ_FT_DRV_10 (3-state), IO8PROG2M25M50M100M_ARSUDQ_FT_DRV_11 (3-state), IO8PROG2M25M50M100M_ARSUDQ_FT_RCV_00 (Input), IO8PROG2M25M50M100M_ARSUDQ_FT_RCV_00_T (Input), IO8PROG2M25M50M100M_ARSUDQ_FT_RCV_01 (Input), IO8PROG2M25M50M100M_ARSUDQ_FT_RCV_01_T (Input), IO8PROG2M25M50M100M_ARSUDQ_FT_RCV_10 (Input), IO8PROG2M25M50M100M_ARSUDQ_FT_RCV_10_T (Input), IO8PROG2M25M50M100M_ARSUDQ_FT_RCV_11 (Input), IO8PROG2M25M50M100M_ARSUDQ_FT_RCV_11_T (Input), IO8PROG2M25M50M100M_ARSUDQ_I2CIN_DRV_00 (3-state), IO8PROG2M25M50M100M_ARSUDQ_I2CIN_DRV_01 (3-state), IO8PROG2M25M50M100M_ARSUDQ_I2CIN_DRV_10 (3-state), IO8PROG2M25M50M100M_ARSUDQ_I2CIN_DRV_11 (3-state), IO8PROG2M25M50M100M_ARWSUDQ_DRV_V33_00 (3-state), IO8PROG2M25M50M100M_ARWSUDQ_DRV_V33_01 (3-state), IO8PROG2M25M50M100M_ARWSUDQ_DRV_V33_10 (3-state), IO8PROG2M25M50M100M_ARWSUDQ_DRV_V33_11 (3-state), IO8PROG2M25M50M100M_ARWSUDQ_FT_DRV_00 (3-state), IO8PROG2M25M50M100M_ARWSUDQ_FT_DRV_01 (3-state), IO8PROG2M25M50M100M_ARWSUDQ_FT_DRV_10 (3-state), IO8PROG2M25M50M100M_ARWSUDQ_FT_DRV_11 (3-state), IO8PROG2M25M50M100M_ARWSUDQ_FT_RCV_00 (Input), IO8PROG2M25M50M100M_ARWSUDQ_FT_RCV_00_T (Input), IO8PROG2M25M50M100M_ARWSUDQ_FT_RCV_01 (Input), IO8PROG2M25M50M100M_ARWSUDQ_FT_RCV_01_T (Input), IO8PROG2M25M50M100M_ARWSUDQ_FT_RCV_10 (Input), IO8PROG2M25M50M100M_ARWSUDQ_FT_RCV_10_T (Input), IO8PROG2M25M50M100M_ARWSUDQ_FT_RCV_11 (Input), IO8PROG2M25M50M100M_ARWSUDQ_FT_RCV_11_T (Input), IO8PROG2M25M50M100M_ARWSUDQ_RCV_V33_0 (Input), IO8PROG2M25M50M100M_ARWSUDQ_RCV_V33_0_T (Input), IO8PROG2M25M50M100M_ARWSUDQ_RCV_V33_1 (Input), IO8PROG2M25M50M100M_ARWSUDQ_RCV_V33_1_T (Input), IO8PROG2M25M50M100M_I2CIN_RCV_ZII2C_00 (Input), IO8PROG2M25M50M100M_I2CIN_RCV_ZII2C_00_T (Input), IO8PROG2M25M50M100M_I2CIN_RCV_ZII2C_01 (Input), IO8PROG2M25M50M100M_I2CIN_RCV_ZII2C_01_T (Input), IO8PROG2M25M50M100M_I2CIN_RCV_ZII2C_10 (Input), IO8PROG2M25M50M100M_I2CIN_RCV_ZII2C_10_T (Input), IO8PROG2M25M50M100M_I2CIN_RCV_ZII2C_11 (Input), IO8PROG2M25M50M100M_I2CIN_RCV_ZII2C_11_T (Input), IO8PROG2M25M50M100M_I2CIN_RCV_ZIV12_0 (Input), IO8PROG2M25M50M100M_I2CIN_RCV_ZIV12_0_T (Input), IO8PROG2M25M50M100M_I2CIN_RCV_ZIV12_1 (Input), IO8PROG2M25M50M100M_I2CIN_RCV_ZIV12_1_T (Input), IO8PROG2M25M50M100M_I2CIN_RCV_ZIV33_0 (Input), IO8PROG2M25M50M100M_I2CIN_RCV_ZIV33_0_T (Input), IO8PROG2M25M50M100M_I2CIN_RCV_ZIV33_1 (Input), IO8PROG2M25M50M100M_I2CIN_RCV_ZIV33_1_T (Input), IO8USB_ID_OTG_FT_DRV_00 (3-state), IO8USB_ID_OTG_FT_DRV_01 (3-state), IO8USB_ID_OTG_FT_DRV_10 (3-state), IO8USB_ID_OTG_FT_DRV_11 (3-state), IO8USB_ID_OTG_FT_RCV_00 (Input), IO8USB_ID_OTG_FT_RCV_00_T (Input), IO8USB_ID_OTG_FT_RCV_01 (Input), IO8USB_ID_OTG_FT_RCV_01_T (Input)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
